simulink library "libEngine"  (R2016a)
settings: Solver=ode45  StartTime=0.0  StopTime=10.0  RelTol=1e-3
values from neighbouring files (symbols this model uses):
  CV = 47000    [initEngine.m]
  IntakeFuelRate = [0.01 0.025 0.04 0.055 0.07 0.085 0.1 0.115 0.13 0.145 0.16]    [initEngine.m]
  TC = 60    [initEngine.m]
  ThrottleValvePosition = [0 10 20 30 40 50 60 70 80 90 100]    [initEngine.m]

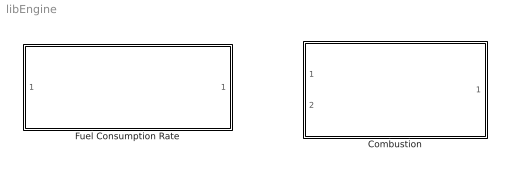
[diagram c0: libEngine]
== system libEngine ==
  Combustion : Subsystem
  Fuel Consumption Rate : Subsystem

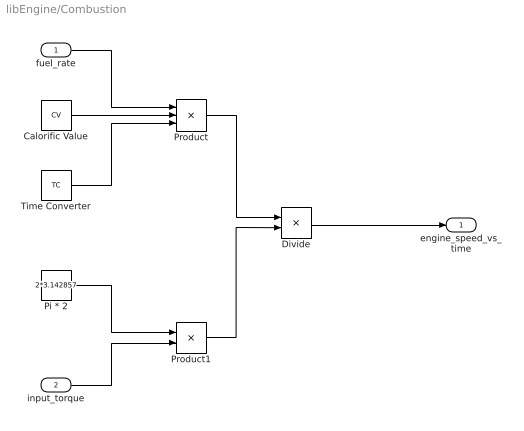
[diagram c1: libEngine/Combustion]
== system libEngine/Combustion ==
  fuel_rate : Inport
  input_torque : Inport  Port=2
  Calorific Value : Constant  Value=CV
  Divide : Product  Inputs=*/
  Pi * 2 : Constant  Value=2*3.142857
  Product : Product  Inputs=3
  Product1 : Product
  Time Converter : Constant  Value=TC
  engine_speed_vs_time : Outport
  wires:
  fuel_rate/1 -> Product/1
  Calorific Value/1 -> Product/2
  Product/1 -> Divide/1
  Pi * 2/1 -> Product1/1
  input_torque/1 -> Product1/2
  Product1/1 -> Divide/2
  Divide/1 -> engine_speed_vs_time/1
  Time Converter/1 -> Product/3

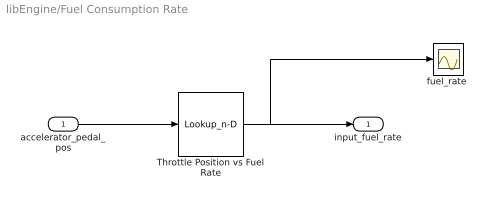
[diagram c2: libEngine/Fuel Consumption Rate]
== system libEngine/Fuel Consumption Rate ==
  accelerator_pedal_pos : Inport
  Throttle Position vs Fuel Rate : Lookup_n-D  NumberOfTableDimensions=1  BreakpointsForDimension1=ThrottleValvePosition  Table=IntakeFuelRate  RndMeth=Simplest
  "fuel_rate " : Scope
  input_fuel_rate : Outport
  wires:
  accelerator_pedal_pos/1 -> Throttle Position vs Fuel Rate/1
  Throttle Position vs Fuel Rate/1 -> input_fuel_rate/1, "fuel_rate "/1
